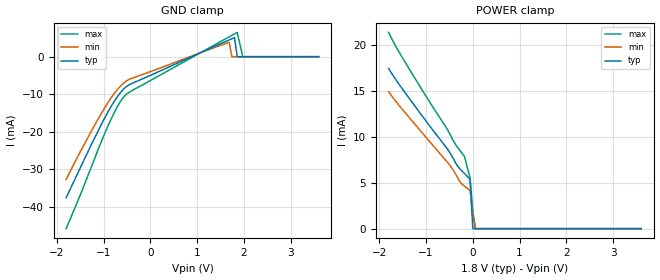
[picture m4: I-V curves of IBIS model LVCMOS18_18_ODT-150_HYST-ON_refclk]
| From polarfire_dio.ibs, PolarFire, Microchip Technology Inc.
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|   Model LVCMOS18_18_ODT-150_HYST-ON_refclk
[Model]   LVCMOS18_18_ODT-150_HYST-ON_refclk
Model_type   Input
Vinl =   0.63
Vinh =   1.17
|   typ   min   max
C_comp   5.210e-12   5.210e-12   5.520e-12
[Temperature Range]  25C   100C   -40C
[Voltage Range]  1.8   1.71   1.89
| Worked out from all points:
|   POWER clamp passes 1 mA (typ) near -0.01 V on its own axis
[GND Clamp]
| Voltage   I(typ)   I(min)   I(max)
-1.8V     -37.55mA   -32.67mA   -45.76mA
-1.358V   -25.93mA   -22.05mA   -32.42mA
-1.063V   -18.41mA   -15.46mA   -23.07mA
-885.9mV  -14.26mA   -11.84mA   -17.91mA
-649.7mV  -9.731mA   -7.982mA   -12.11mA
-472.5mV  -7.621mA   -6.177mA   -9.637mA
1.688V    4.466mA    3.822mA    5.297mA
1.744V    4.771mA    0A         5.681mA
1.8V      5.074mA    0A         6.065mA
1.859V    0A         0A         6.467mA
1.977V    0A         0A         0A
3.6V      0A         0A         0A
[POWER Clamp]
| Voltage   I(typ)   I(min)   I(max)
-1.8V     17.49mA    14.96mA    21.42mA
-1.654V   16.31mA    13.95mA    19.96mA
-1.299V   13.8mA     11.76mA    16.92mA
-531.6mV  8.608mA    7.172mA    10.71mA
-354.4mV  7.053mA    5.853mA    9.061mA
-295.3mV  6.629mA    5.275mA    8.665mA
-236.2mV  6.324mA    4.864mA    8.27mA
-177.2mV  6.016mA    4.637mA    7.874mA
-59.06mV  5.391mA    4.164mA    5.537mA
0V        0A         1.624mA    1.903mA
56.25mV   0A         0A         0A
3.6V      0A         0A         0A
